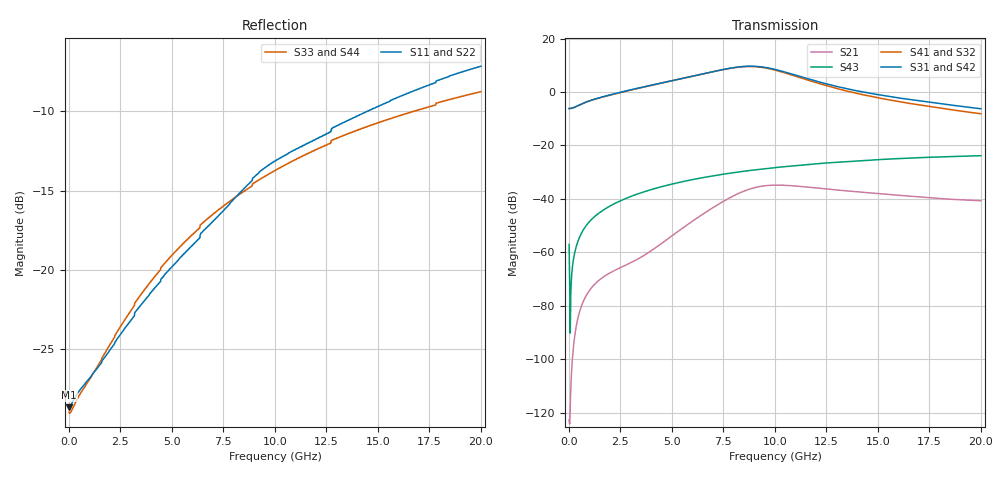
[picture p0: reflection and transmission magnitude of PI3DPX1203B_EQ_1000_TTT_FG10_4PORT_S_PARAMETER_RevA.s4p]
! NPort=4 DATA=2000 NOISE=0 GROUPDELAY=0 COMPLEX_DATAFORMAT=POLAR
! NumOfBlock=1 NumOfParam=0
! .MODEL Smodel S TSTONEFILE=PI3DPX1203B_EQ_1000_TTT_FG10_4PORT_S_PARAMETER_RevA.s4p TYPE=S
!  -- The above .MODEL line can be used for the S element in the netlist.
! The s parameter is extracted from the linear redriver, it is not bi-directional; only s(4,1)s(4,2) and s(3,1)s(3,2)
! should be the insertion loss
!Port definition:
!Port1 = input+
!Port2 = input-
!Port3 = output+
!Port4 = output-
# Hz S MA R  50
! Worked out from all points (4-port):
!   2000 points, 10 MHz to 20 GHz, reference 50 ohm
!   strongest paths, dB at 10 MHz, 5.01 GHz, 10.01 GHz, 15.01 GHz, 20 GHz:
!     S31: -6.2, 4.3, 8.5, -1.0, -6.2
!     S42: -6.2, 4.3, 8.5, -1.0, -6.2
!     S41: -6.2, 4.2, 8.2, -2.2, -8.1
!     S32: -6.2, 4.2, 8.2, -2.2, -8.1
!     S43: -57.1, -34.4, -28.3, -25.3, -23.8
!     S21: -122.7, -53.8, -34.8, -38.0, -40.7
!   lowest |S11| = -28.6 dB at 10 MHz (marker M1), VSWR 1.08, Z = 46.4 - j0.0306 ohm
!   |S11| at or under -10 dB: start of sweep to 14.53 GHz
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1e7  0.03701 -179.5  7.338e-07 10.6  0 0.0  0 0.0
     7.338e-07 10.6  0.03701 -179.5  0 0.0  0 0.0
     0.4917 -0.1  0.4917 179.9  0.03566 178.2  0.001403 -77.8
     0.4917 179.9  0.4917 -0.1  0.001403 -77.8  0.03566 178.2
3.12e9  0.07102 -126.6  0.0006742 130.3  1.666e-10 55.8  2.785e-09 107.0
        0.0006739 130.3  0.07102 -126.6  2.785e-09 107.0  1.666e-10 55.8
        1.13 -2.1  1.117 179.2  0.07625 -126.4  0.01154 77.6
        1.117 179.2  1.13 -2.1  0.01154 77.6  0.07625 -126.4
5.97e9  0.1189 -110.9  0.00376 149.8  1.452e-08 -119.5  1.3e-07 67.7
        0.00376 149.8  0.1189 -110.9  1.3e-07 67.7  1.453e-08 -119.4
        1.97 -42.1  1.968 139.6  0.1289 -117.1  0.02286 65.3
        1.968 139.6  1.97 -42.1  0.02286 65.3  0.1289 -117.1
8.36e9  0.1768 -105.3  0.01329 109.7  3.503e-07 156.3  9.689e-07 18.3
        0.01328 109.7  0.1768 -105.3  9.679e-07 18.3  3.505e-07 156.3
        2.993 -99.7  2.962 81.7  0.1743 -115.9  0.03242 53.1
        2.963 81.7  2.992 -99.7  0.03242 53.1  0.1743 -115.9
9.86e9  0.2173 -107.2  0.01805 66.4  1.154e-06 95.1  1.962e-06 -19.2
        0.01804 66.5  0.2173 -107.2  1.96e-06 -19.1  1.155e-06 95.1
        2.737 -148.8  2.665 32.4  0.203 -116.2  0.03799 45.1
        2.667 32.4  2.736 -148.8  0.03799 45.1  0.203 -116.2
1.205e10  0.2592 -109.1  0.016 24.9  2.959e-06 29.8  3.711e-06 -47.2
          0.01597 25.0  0.2592 -109.1  3.711e-06 -47.0  2.961e-06 29.9
          1.584 164.0  1.482 -14.5  0.2398 -117.5  0.04562 34.0
          1.483 -14.5  1.583 164.0  0.04562 34.0  0.2398 -117.5
2e10  0.4376 -117.3  0.009183 -17.9  2.226e-05 -108.3  3.168e-05 -133.9
      0.009226 -17.6  0.4377 -117.3  3.176e-05 -133.8  2.229e-05 -108.3
      0.4872 77.5  0.3931 -88.5  0.3637 -123.9  0.06431 -7.1
      0.3928 -88.7  0.4879 77.5  0.06431 -7.1  0.3637 -123.9
